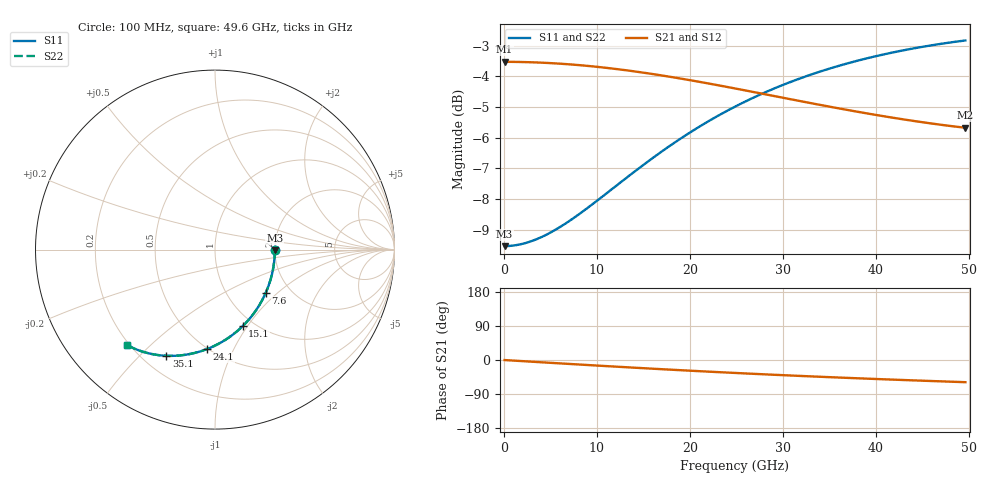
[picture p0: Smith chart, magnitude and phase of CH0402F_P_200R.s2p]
# GHz S RI R 200
! S-Parameters data
! Freq  reS11  imS11  reS21  imS21  reS12  imS12  reS22  imS22
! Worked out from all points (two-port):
!   100 points, 100 MHz to 49.6 GHz, reference 200 ohm
!   highest |S21| = -3.52 dB at 100 MHz (marker M1); lowest = -5.7 dB at 49.6 GHz (marker M2)
!   |S21| within 3 dB of the highest: start of sweep to end of sweep
!   lowest |S11| = -9.5 dB at 100 MHz (marker M3), VSWR 2.00, Z = 400 - j2.97 ohm
!   |S11| at or under -10 dB: nowhere
!   |S22| runs from -9.5 to -2.8 dB; largest |S21 - S12| = 0
!   S11 on the Smith chart (normalised r, x): 100 MHz: 2.00, -0.01; 7.6 GHz: 1.51, -0.84; 15.1 GHz: 0.88, -0.95; 24.1 GHz: 0.50, -0.79; 35.1 GHz: 0.29, -0.60; 49.6 GHz: 0.19, -0.43
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0.1  0.3333 -0.0033  0.6667 -0.00172  0.6667 -0.00172  0.3333 -0.0033
1.6  0.331 -0.0527  0.6658 -0.0276  0.6658 -0.0276  0.331 -0.0527
3.6  0.3216 -0.1178  0.6621 -0.0617  0.6621 -0.0617  0.3216 -0.1178
5.6  0.3053 -0.1808  0.6558 -0.0953  0.6558 -0.0953  0.3053 -0.1808
7.6  0.2827 -0.2407  0.6469 -0.1278  0.6469 -0.1278  0.2827 -0.2407
8.6  0.2692 -0.2693  0.6415 -0.1437  0.6415 -0.1437  0.2692 -0.2693
12.1  0.2122 -0.3606  0.6185 -0.1961  0.6185 -0.1961  0.2122 -0.3606
15.1  0.1539 -0.4266  0.5943 -0.2369  0.5943 -0.2369  0.1539 -0.4266
16.6  0.1225 -0.4551  0.581 -0.2556  0.581 -0.2556  0.1225 -0.4551
18.1  0.0901 -0.4806  0.567 -0.2732  0.567 -0.2732  0.0901 -0.4806
20.1  0.0459 -0.51  0.5475 -0.2949  0.5475 -0.2949  0.0459 -0.51
22.1  0.00106 -0.5343  0.5274 -0.3147  0.5274 -0.3147  0.00106 -0.5343
24.1  -0.0437 -0.5538  0.5069 -0.3324  0.5069 -0.3324  -0.0437 -0.5538
25.1  -0.0659 -0.5619  0.4965 -0.3406  0.4965 -0.3406  -0.0659 -0.5619
27.1  -0.1096 -0.5748  0.4758 -0.3557  0.4758 -0.3557  -0.1096 -0.5748
29.1  -0.1522 -0.5839  0.4552 -0.3691  0.4552 -0.3691  -0.1522 -0.5839
33.1  -0.2329 -0.5919  0.4149 -0.3914  0.4149 -0.3914  -0.2329 -0.5919
35.1  -0.2707 -0.5916  0.3954 -0.4006  0.3954 -0.4006  -0.2707 -0.5916
38.1  -0.3239 -0.5865  0.3672 -0.4125  0.3672 -0.4125  -0.3239 -0.5865
41.6  -0.3805 -0.5751  0.336 -0.424  0.336 -0.424  -0.3805 -0.5751
45.6  -0.4381 -0.5561  0.3026 -0.4347  0.3026 -0.4347  -0.4381 -0.5561
49.6  -0.4884 -0.5324  0.2715 -0.4438  0.2715 -0.4438  -0.4884 -0.5324
